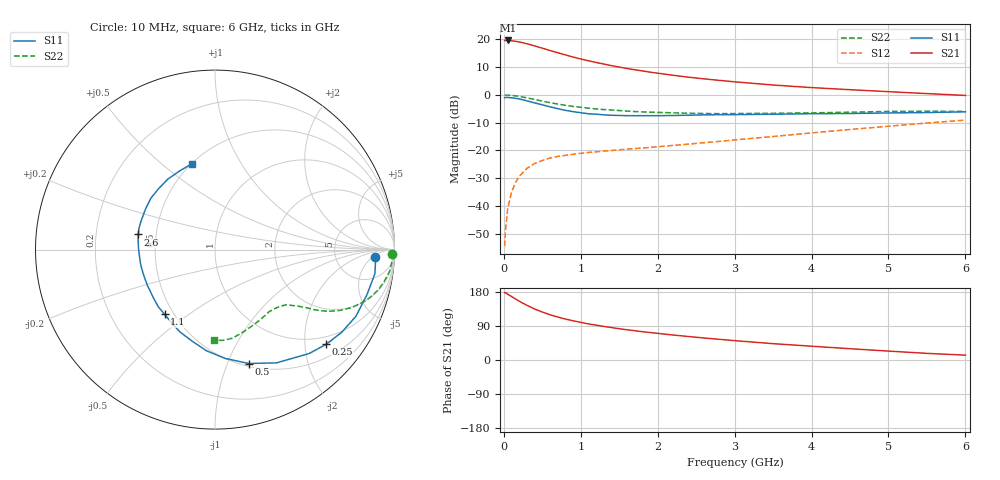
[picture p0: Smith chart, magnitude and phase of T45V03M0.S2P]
! Infineon Technologies  Discrete & RF Semiconductors
! BFR182T
! Si NPN RF Bipolar Junction Transistor in SC75
! VCE = 5 V  IC = 3 mA
! Common Emitter S-Parameters:  October  1999
# GHz  S  MA  R  50
!  f  S11  S21  S12  S22
! GHz  MAG  ANG  MAG  ANG  MAG  ANG  MAG  ANG
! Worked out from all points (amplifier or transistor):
!   36 points, 10 MHz to 6 GHz, reference 50 ohm
!   highest |S21| = 19.6 dB at 50 MHz (marker M1)
!   |S21| within 3 dB of that: start of sweep to 526.6 MHz
!   unconditionally stable (mu >= 1): 1.759 GHz to 4.225 GHz
!   at 250 MHz: K = 0.19, MSG = 23.3 dB, |S12| = -27.9 dB
!   at 1.4 GHz: K = 0.88, MSG = 15.3 dB, |S12| = -20.0 dB
!   at 6 GHz: K = 0.83, MSG = 4.4 dB, |S12| = -9.1 dB
!   lowest NFmin = 1.10 dB at 450 MHz
!   S11 on the Smith chart (normalised r, x): 10 MHz: 15, -6; 250 MHz: 0.80, -2.50; 500 MHz: 0.53, -1.20; 1.1 GHz: 0.45, -0.41; 2.6 GHz: 0.40, +0.08; 6 GHz: 0.50, +0.64
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0.01  0.891 -2.8  9.513 177.9  0.0019 75.5  0.987 -1.4
0.02  0.8965 -2.0  9.448 177.7  0.0034 108.4  0.9895 -1.5
0.05  0.901 -8.6  9.516 173.6  0.009 85.4  0.9895 -3.7
0.1  0.8832 -16.5  9.381 167.6  0.0178 83.5  0.9794 -7.2
0.15  0.8686 -25.3  9.208 161.2  0.0263 76.4  0.9603 -10.5
0.2  0.8435 -33.0  8.951 155.3  0.0342 74.4  0.9387 -13.6
0.25  0.814 -40.4  8.635 149.7  0.0405 68.9  0.912 -16.4
0.3  0.7809 -47.9  8.293 144.3  0.0476 66.0  0.885 -18.9
0.4  0.718 -61.5  7.608 134.6  0.0585 60.3  0.826 -23.1
0.5  0.662 -73.5  6.914 126.6  0.0659 55.4  0.7731 -26.0
0.6  0.6087 -84.7  6.271 119.4  0.0733 52.5  0.7246 -28.3
0.8  0.526 -104.0  5.234 108.1  0.0817 48.5  0.6493 -31.1
0.9  0.499 -112.9  4.789 103.5  0.0853 47.7  0.6192 -32.0
1.1  0.457 -127.9  4.107 95.2  0.0922 46.6  0.5763 -33.6
1.3  0.4371 -141.2  3.583 88.6  0.0976 46.4  0.5436 -35.1
1.6  0.4228 -157.7  2.984 79.8  0.1056 47.8  0.5103 -37.0
2.2  0.4257 179.9  2.252 65.9  0.1232 51.9  0.4753 -42.5
2.6  0.4362 168.8  1.941 58.1  0.1378 54.6  0.4621 -47.1
3.5  0.4482 149.8  1.503 43.1  0.1782 58.4  0.466 -58.3
4.5  0.4624 132.9  1.238 29.8  0.2383 58.7  0.4874 -72.1
5.5  0.4808 114.1  1.054 17.5  0.3117 55.7  0.5076 -85.2
6  0.4957 104.9  0.977 12.8  0.3516 52.7  0.5052 -90.9
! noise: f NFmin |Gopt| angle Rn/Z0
0.45  1.1  0.37  30  0.33
0.9  1.2  0.35  61  0.26
1.8  1.85  0.27  133  0.2
